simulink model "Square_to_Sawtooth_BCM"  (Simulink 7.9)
settings: Solver=ode45  StartTime=0.0  StopTime=10.0  RelTol=1e-3
undefined symbols (not defined in the file or in its folder): sigbuilder_block
libraries: nesl_utility x6, fl_lib x5, Memristor_lib x2

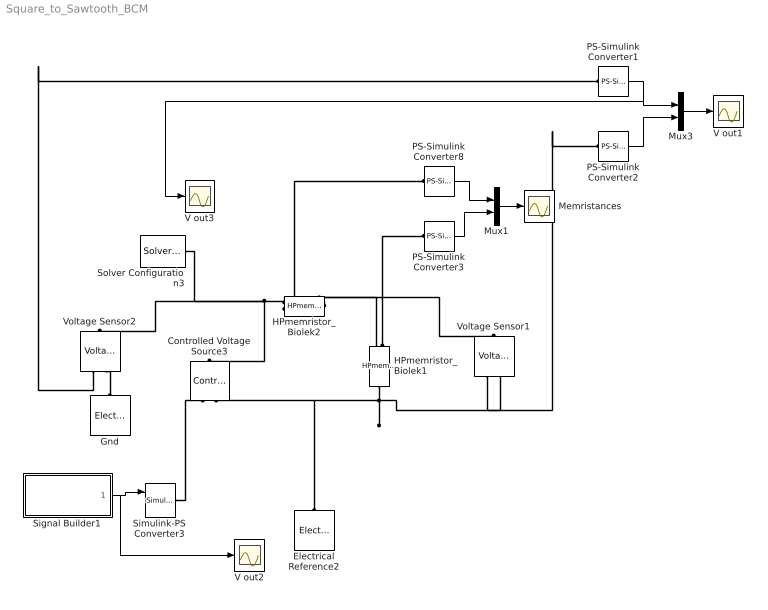
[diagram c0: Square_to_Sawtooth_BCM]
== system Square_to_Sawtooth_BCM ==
  Controlled Voltage Source3 : fl_lib/Electrical/Electrical Sources/Controlled Voltage Source  i_Log=off  v_Log=off  LocalVarNames=|i|v  LocalVarDescs=|i|v  LocalVarLogging=[0 0]
  Electrical Reference2 : fl_lib/Electrical/Electrical Elements/Electrical Reference  i_Log=off  LocalVarNames=|i  LocalVarDescs=|i  LocalVarLogging=0
  Gnd : fl_lib/Electrical/Electrical Elements/Electrical Reference  i_Log=off  LocalVarNames=|i  LocalVarDescs=|i  LocalVarLogging=0
  HPmemristor_Biolek1 : Memristor_lib/HPmemristor_Biolek  R_off=20 kOhm  R_on=20 Ohm  pp=10 m  u_v=1e-13 m^2/s/V  D=1e-8 m  w0=9.89e-9 m  i_Log=off  v_Log=off  w_Log=off  F_Log=off  M_Log=off  LocalVarNames=|i|v|w|F|M  LocalVarDescs=|i|v|w|F|M  LocalVarLogging=[0 0 0 0 0]
  HPmemristor_Biolek2 : Memristor_lib/HPmemristor_Biolek  R_off=20 kOhm  R_on=20 Ohm  pp=10 m  u_v=1e-13 m^2/s/V  D=1e-8 m  w0=.01e-9 m  i_Log=off  v_Log=off  w_Log=off  F_Log=off  M_Log=off  LocalVarNames=|i|v|w|F|M  LocalVarDescs=|i|v|w|F|M  LocalVarLogging=[0 0 0 0 0]
  Memristances : Scope
  Mux1 : Mux  Inputs=2
  Mux3 : Mux  Inputs=2
  PS-Simulink Converter{1..3,8} (4 alike) : nesl_utility/PS-Simulink Converter  PhysicalDomain=network_engine_domain  LeftPortType=input  RightPortType=output  SubClassName=ps_output  Unit=1  AffineConversion=off
  Signal Builder1 : Subsystem  Tag=STV Subsys  LoadFcn=sigbuilder_block('load');  StartFcn=sigbuilder_block('start');  StopFcn=sigbuilder_block('stop');  ClipboardFcn=sigbuilder_block('clipboard');
  Simulink-PS Converter3 : nesl_utility/Simulink-PS Converter  PhysicalDomain=network_engine_domain  LeftPortType=input  RightPortType=output  SubClassName=ps_input  Unit=1  AffineConversion=off  InputFilterTimeConstant=.001  UdotUserProvided=2  SimscapeFilterOrder=1  InputFiltering=derivs
  Solver Configuration3 : nesl_utility/Solver Configuration  PhysicalDomain=network_engine_domain  LeftPortType=input  RightPortType=generic  SubClassName=solver  UseCustomDae=off  DoDC=off  ResidualTolerance=1e-9  UseLocalSolver=off  LocalSolverChoice=NE_BACKWARD_EULER_ADVANCER  LocalSolverSampleTime=.001  DoFixedCost=off  MaxNonlinIter=3  MaxModeIter=2  LinearAlgebra=Sparse  Accelerate=off  Profile=off  UseLocalSampling=off  DelaysMemoryBudget=1024
  V out1 : Scope
  V out2 : Scope
  V out3 : Scope
  Voltage Sensor1 : fl_lib/Electrical/Electrical Sensors/Voltage Sensor  i1_Log=off  v1_Log=off  LocalVarNames=|i1|v1  LocalVarDescs=|i1|v1  LocalVarLogging=[0 0]
  Voltage Sensor2 : fl_lib/Electrical/Electrical Sensors/Voltage Sensor  i1_Log=off  v1_Log=off  LocalVarNames=|i1|v1  LocalVarDescs=|i1|v1  LocalVarLogging=[0 0]
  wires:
  Signal Builder1/1(Signal 3) -> Simulink-PS Converter3/1, V out2/1
  Mux3/1 -> V out1/1
  Mux1/1 -> Memristances/1
  PS-Simulink Converter8/1 -> Mux1/1
  PS-Simulink Converter1/1 -> Mux3/1, V out3/1
  PS-Simulink Converter2/1 -> Mux3/2
  PS-Simulink Converter3/1 -> Mux1/2
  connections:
  HPmemristor_Biolek2/RConn1 -- Voltage Sensor1/LConn1 -- HPmemristor_Biolek1/RConn1
  HPmemristor_Biolek2/LConn1 -- Solver Configuration3/RConn1 -- Controlled Voltage Source3/LConn1 -- Voltage Sensor2/LConn1
  HPmemristor_Biolek1/LConn1 -- Voltage Sensor1/RConn2 -- Controlled Voltage Source3/RConn2 -- Electrical Reference2/LConn1
  HPmemristor_Biolek2/RConn2 -- PS-Simulink Converter8/LConn1
  HPmemristor_Biolek1/RConn2 -- PS-Simulink Converter3/LConn1
  Voltage Sensor1/RConn1 -- PS-Simulink Converter2/LConn1
  Simulink-PS Converter3/RConn1 -- Controlled Voltage Source3/RConn1
  Gnd/LConn1 -- Voltage Sensor2/RConn2
  Voltage Sensor2/RConn1 -- PS-Simulink Converter1/LConn1

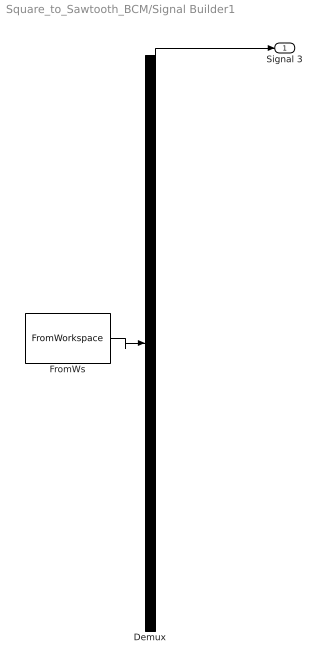
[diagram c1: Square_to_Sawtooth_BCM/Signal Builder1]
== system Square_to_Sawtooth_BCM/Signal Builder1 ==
  Demux : Demux  Tag=STV Demux  Outputs=1
  FromWs : FromWorkspace  Tag=STV FromWs  VariableName=tuvar  SampleTime=0  SigBuilderData=DataTag0  VnvData=DataTag1
  Signal 3 : Outport  Tag=STV Outport
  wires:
  FromWs/1 -> Demux/1
  Demux/1 -> Signal 3/1
